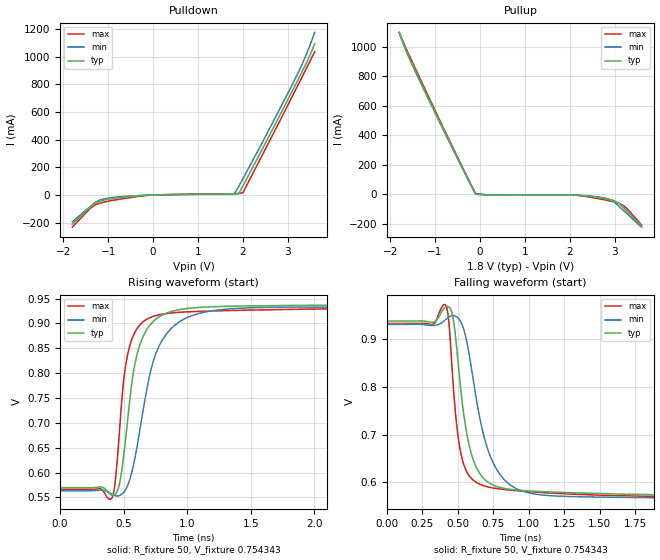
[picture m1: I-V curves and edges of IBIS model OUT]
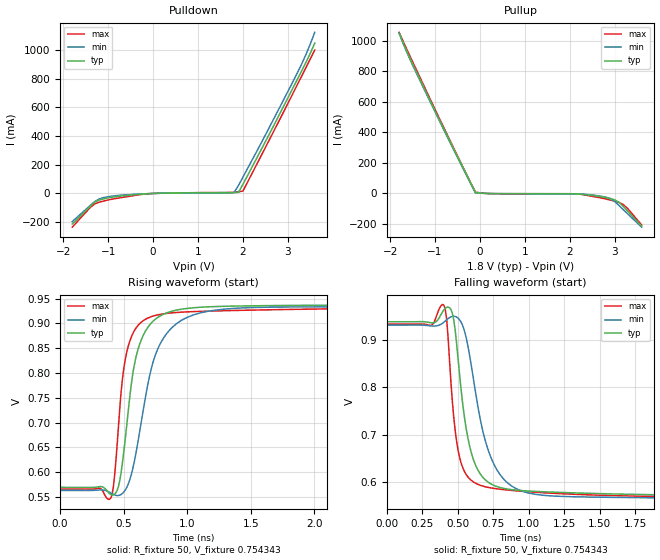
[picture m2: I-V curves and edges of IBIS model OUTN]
|   IBIS File of SG2520VGN E
|   LVDS, Vcc=1.8V, Io=3.5mA, fo>212.5MHz
[IBIS Ver]   3.2
[File Name]   sg2520vgn_hf_35m_18v.ibs
[File Rev]   1.0
[Date]   July 22, 2020
[Source]
Fairchild Ensigna Lab's Method
[Notes]
Created by Minoru Kozaki
[Disclaimer]
Seiko Epson Corporation makes no warranty with respect to the
information contained herein.
[Copyright]
Copyright(C) 2020, Seiko Epson Corporation. All rights reserved.
|   Component
[Component]   SG2520VGN
[Manufacturer]  Seiko Epson Corporation
[Package]
R_pkg   17.7m   NA   NA
L_pkg   235p   NA   NA
C_pkg   208f   NA   NA
[Pin]   signal_name   model_name   R_pin   L_pin   C_pin
1   OE/ST   NC
2   NC   NC
3   GND   GND
4   OUT   OUT   17.7m   235p   208f
5   OUTN   OUTN   10.4m   129p   221f
6   VCC   POWER
[Diff Pin] inv_pin  vdiff  tdelay_typ
4   5   0   0
| Models and submodels in the file (2): OUT (Output), OUTN (Output)
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|   Model OUT
[Model]   OUT
Model_type   Output
Polarity   Non-Inverting
Vref = 0.75
Vmeas = 0.75
Rref = 50
Cref = 0
C_comp   4.5p   4.5p   4.5p
[Temperature Range]   25   105   -40
[Voltage Range]   1.8   1.71   1.89
[Pullup Reference]   1.8   1.71   1.89
[Pulldown Reference]   0   0   0
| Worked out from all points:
|   slope of the pulldown table from 0 to 0.27 V, typ, clamps not added: 120 ohm
|   slope of the pullup table from 0 to 0.27 V, typ, clamps not added: 79.1 ohm
|   falling waveform, R_fixture 50, V_fixture 0.754343: 20-80 % time 115ps typ, 169ps min, 84.1ps max; typ from 0.938 V to 0.57 V
|   rising waveform, R_fixture 50, V_fixture 0.754343: 20-80 % time 133ps typ, 191ps min, 99.3ps max; typ from 0.57 V to 0.938 V
[Pullup]
-1.8V     1.091A     1.097A     1.096A
-1.6V     942.8mA    938.8mA    957.1mA
-1.4V     812.5mA    804.6mA    827mA
-700mV    369.6mA    364.9mA    378.6mA
-100mV    2.668mA    1.663mA    6.415mA
300mV     -3.335mA   -3.001mA   -3.333mA
2.1V      -4.376mA   -4.506mA   -4.182mA
2.8V      -28.36mA   -25.79mA   -37.62mA
3V        -43.54mA   -54.45mA   -52mA
3.1V      -60.94mA   -81.52mA   -60.73mA
3.2V      -89.46mA   -109.4mA   -75.76mA
3.6V      -213.9mA   -220.9mA   -206.8mA
[Pulldown]
-1.8V     -211.3mA   -194mA     -232.6mA
-1.4V     -87.54mA   -82.93mA   -96.92mA
-1.3V     -60.52mA   -56.17mA   -72.49mA
-1.2V     -45mA      -37.88mA   -60.28mA
-1V       -30.83mA   -22.63mA   -45.07mA
-100mV    -1.55mA    -1.238mA   -1.808mA
1.8V      5.997mA    5.208mA    7.922mA
1.9V      7.357mA    57.29mA    11.53mA
2V        65.7mA     117.4mA    16.91mA
3.2V      816.1mA    863.5mA    777.9mA
3.4V      945.5mA    1.006A     906.5mA
3.6V      1.093A     1.176A     1.037A
[Falling Waveform]
R_fixture = 50
V_fixture = 0.754343
V_fixture_min = 0.747368
V_fixture_max = 0.750213
0s        938.4mV    931.4mV    933.4mV
410ps     967.3mV    940.7mV    973.2mV
430ps     969mV      945.7mV    952.7mV
460ps     953.2mV    949.8mV    831.7mV
520ps     793.8mV    936.9mV    661.1mV
590ps     664.4mV    848.7mV    609.4mV
690ps     605.3mV    688.7mV    591.7mV
820ps     587.2mV    607.3mV    584.8mV
1.05ns    580.6mV    574.6mV    579mV
4ns       570mV      563.9mV    566.6mV
[Rising Waveform]
R_fixture = 50
V_fixture = 0.754343
V_fixture_min = 0.747368
V_fixture_max = 0.750213
0s        569.7mV    563.4mV    566.4mV
400ps     555.2mV    558mV      546.7mV
450ps     562.8mV    552.9mV    626.2mV
500ps     633.6mV    560.2mV    785.4mV
540ps     726.5mV    579.7mV    847.1mV
610ps     842.4mV    659.1mV    891.5mV
730ps     903.3mV    821.1mV    914mV
900ps     925.7mV    895.9mV    921.7mV
1.2ns     933.7mV    925.7mV    925.1mV
4ns       938.2mV    931.7mV    932.8mV
[Ramp]
R_load = 50
dV/dt_r   0.22109/133.77p   0.21984/189.39p   0.22055/100.11p
dV/dt_f   0.22109/115.12p   0.21984/168.16p   0.22055/84.04p
|   Model OUTN
[Model]   OUTN
Model_type   Output
Polarity   Inverting
Vref = 0.75
Vmeas = 0.75
Rref = 50
Cref = 0
C_comp   4.5p   4.5p   4.5p
[Temperature Range]   25   105   -40
[Voltage Range]   1.8   1.71   1.89
[Pullup Reference]   1.8   1.71   1.89
[Pulldown Reference]   0   0   0
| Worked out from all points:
|   slope of the pulldown table from 0 to 0.27 V, typ, clamps not added: 120 ohm
|   slope of the pullup table from 0 to 0.27 V, typ, clamps not added: 79 ohm
|   falling waveform, R_fixture 50, V_fixture 0.754343: 20-80 % time 115ps typ, 167ps min, 83.3ps max; typ from 0.938 V to 0.57 V
|   rising waveform, R_fixture 50, V_fixture 0.754343: 20-80 % time 133ps typ, 191ps min, 98.4ps max; typ from 0.57 V to 0.938 V
[Pullup]
-1.8V     1.046A     1.049A     1.054A
-1.6V     909mA      903.6mA    923.5mA
-1.4V     784.2mA    776.4mA    798.2mA
-800mV    416.4mA    411.8mA    426.1mA
-100mV    2.672mA    1.666mA    6.416mA
200mV     -2.75mA    -2.256mA   -2.854mA
2.1V      -4.376mA   -4.509mA   -4.181mA
2.8V      -28.69mA   -26.03mA   -38mA
3V        -43.96mA   -54.83mA   -52.59mA
3.1V      -61.37mA   -82.17mA   -61.37mA
3.2V      -90.12mA   -110.3mA   -76.28mA
3.6V      -215.9mA   -222.8mA   -208.4mA
[Pulldown]
-1.8V     -213.6mA   -196mA     -235mA
-1.4V     -88.43mA   -83.78mA   -97.72mA
-1.3V     -61.04mA   -56.68mA   -73.02mA
-1.2V     -45.35mA   -38.15mA   -60.71mA
-1V       -31.04mA   -22.76mA   -45.36mA
-100mV    -1.552mA   -1.24mA    -1.811mA
1.8V      5.998mA    5.209mA    7.92mA
1.9V      7.354mA    55.34mA    11.51mA
2V        63.47mA    113.4mA    16.56mA
3.2V      787.7mA    832.7mA    750.8mA
3.4V      911.7mA    966mA      875mA
3.6V      1.048A     1.123A     1A
[Falling Waveform]
R_fixture = 50
V_fixture = 0.754343
V_fixture_min = 0.747368
V_fixture_max = 0.750213
0s        938.5mV    931.5mV    933.4mV
400ps     963.4mV    937.4mV    973.9mV
420ps     968.9mV    942.6mV    944.7mV
450ps     964.7mV    948.8mV    812.7mV
520ps     801.3mV    938.7mV    642.8mV
580ps     679mV      871.3mV    607.8mV
670ps     612.2mV    714.7mV    592.3mV
800ps     588.5mV    614.7mV    585.1mV
1.05ns    580.5mV    574.2mV    578.7mV
4ns       570mV      563.9mV    566.5mV
[Rising Waveform]
R_fixture = 50
V_fixture = 0.754343
V_fixture_min = 0.747368
V_fixture_max = 0.750213
0s        569.6mV    563.4mV    566.3mV
390ps     556.7mV    559.7mV    545.6mV
440ps     559.3mV    553.4mV    626.6mV
490ps     618.4mV    557.3mV    787.3mV
530ps     708.6mV    572.6mV    848.2mV
600ps     835.3mV    643mV      891.7mV
720ps     901.5mV    811.3mV    913.9mV
880ps     924.7mV    891.5mV    921.3mV
1.2ns     933.8mV    926.1mV    925.1mV
4ns       938.2mV    931.9mV    932.8mV
[Ramp]
R_load = 50
dV/dt_r   0.22087/133.22p   0.21963/188.12p   0.22032/99.09p
dV/dt_f   0.22087/114.09p   0.21963/166.16p   0.22032/82.93p
